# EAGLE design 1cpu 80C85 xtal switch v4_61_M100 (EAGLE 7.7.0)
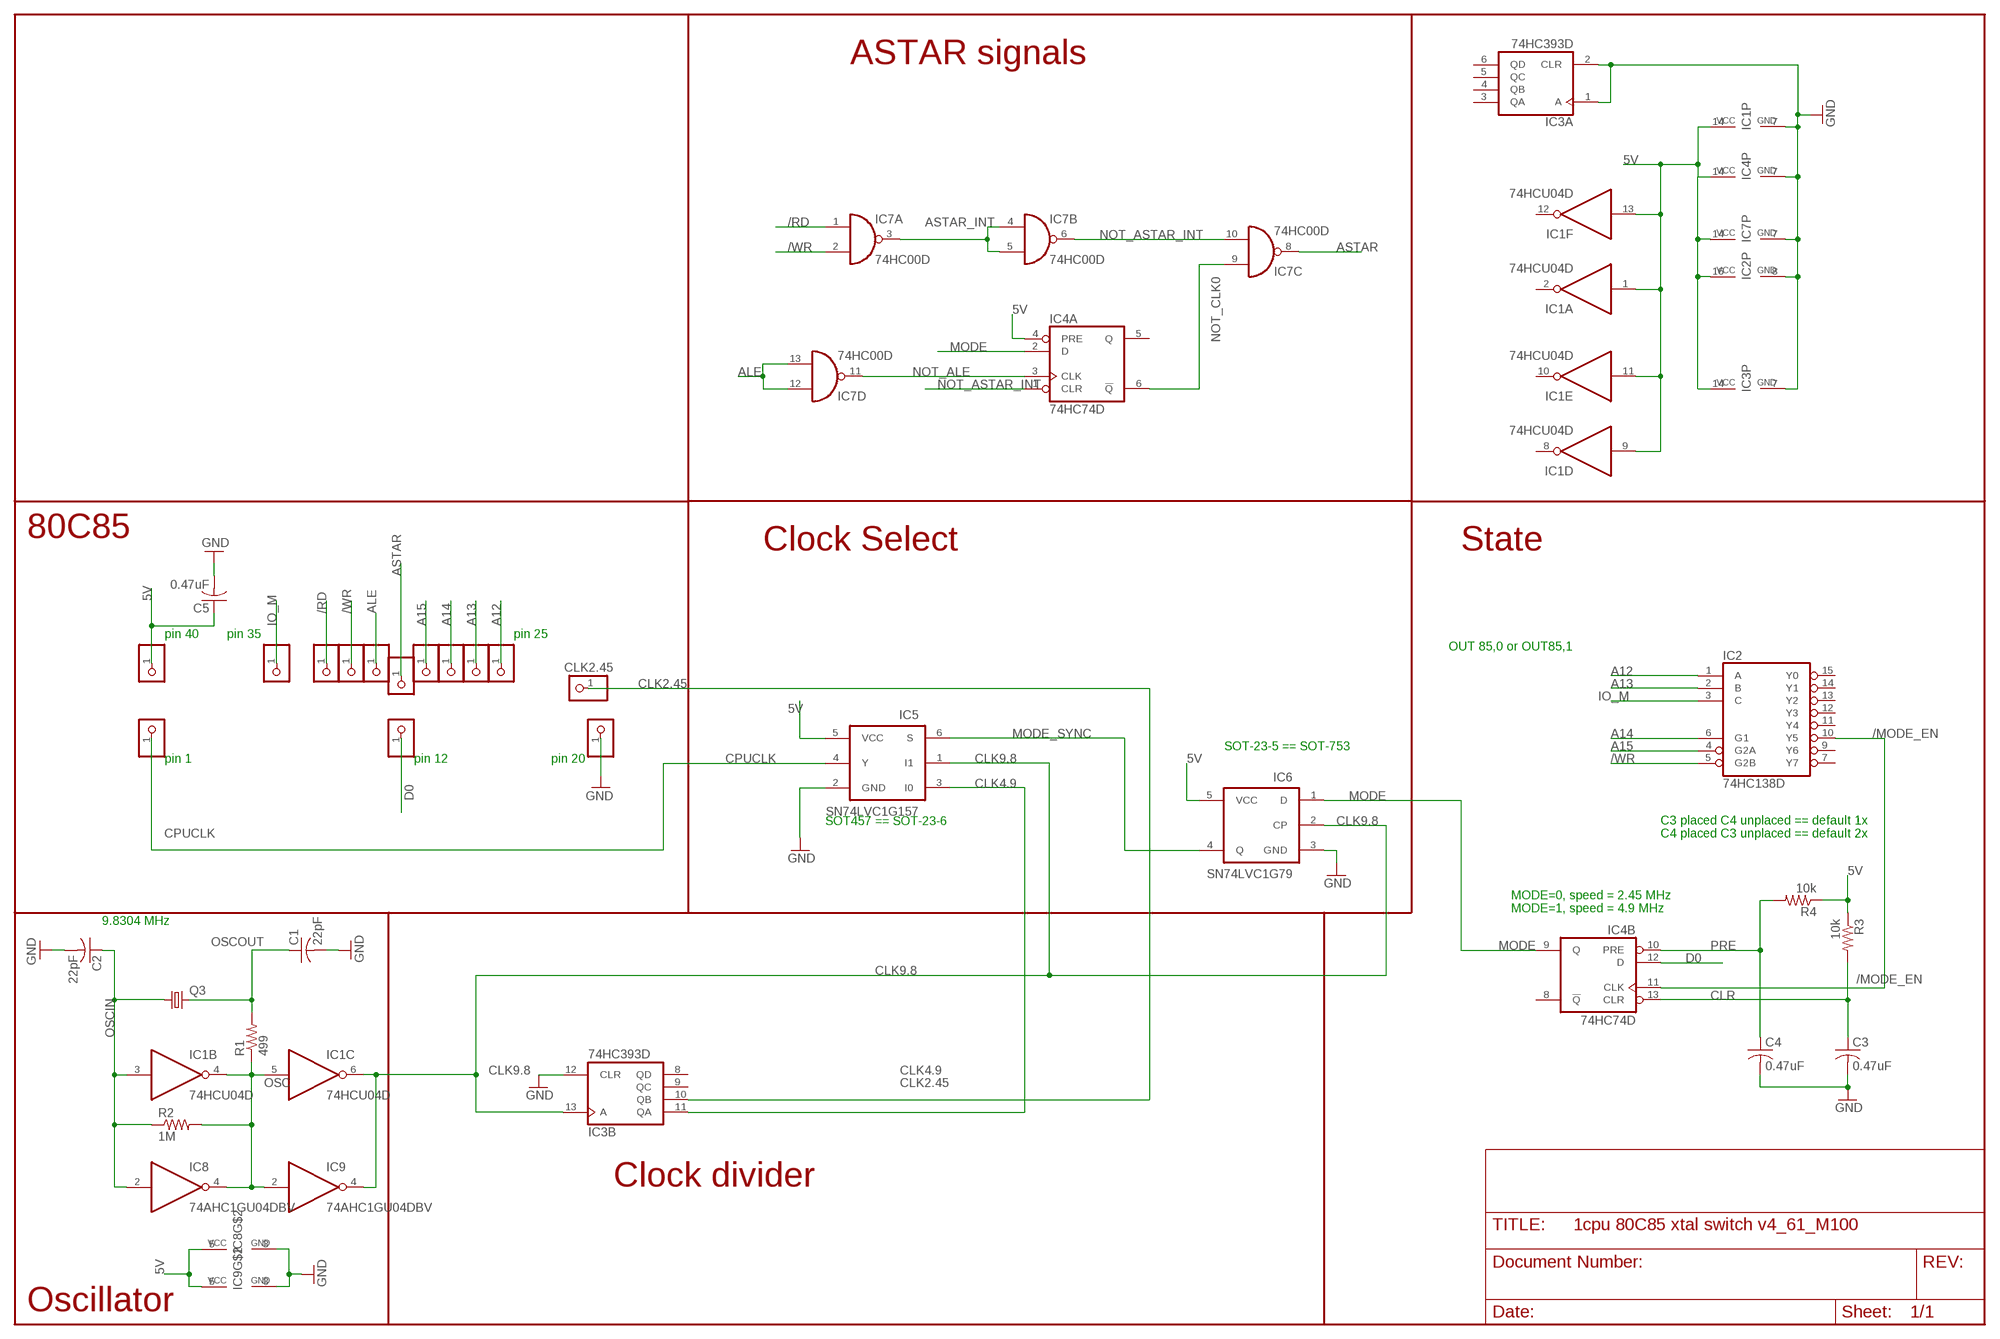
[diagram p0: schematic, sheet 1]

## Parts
5V  PINHD-1X1  [1X01]
5V1  PINHD-1X1  [1X01]
5V2  PINHD-1X1  [1X01]
5V3  PINHD-1X1  [1X01]
5V5  PINHD-1X1  [1X01]
5V7  PINHD-1X1  [1X01]
5V8  PINHD-1X1  [1X01]
5V9  PINHD-1X1  [1X01]
5V10  PINHD-1X1  [1X01]
C1  22pF  C-US025-025X050  [C025-025X050]
C2  22pF  C-US025-025X050  [C025-025X050]
C3  0.47uF  C-US025-025X050  [C025-025X050]
C4  0.47uF  C-US025-025X050  [C025-025X050]
C5  0.47uF  C-US025-025X050  [C025-025X050]
GND5  PINHD-1X1  [1X01]
GND8  PINHD-1X1  [1X01]
GND10  PINHD-1X1  [1X01]
IC1  74HCU04D  74HC04D  [SO14]
IC2  74HC138D  [SO16]
IC3  74HC393D  [SO14]
IC4  74HC74D  [SO14]
IC5  SN74LVC1G157  [SOT23-6]
IC6  SN74LVC1G79  [SOT23-5]
IC7  74HC00D  [SO14]
IC8  74AHC1GU04DBV  [SOT23-5]
IC9  74AHC1GU04DBV  [SOT23-5]
Q3  CRYSTALHC49S  [HC49/S]
R1  499  R-US_0204/5  [0204/5]
R2  1M  R-US_0204/5  [0204/5]
R3  10k  R-US_0204/5  [0204/5]
R4  10k  R-US_0204/5  [0204/5]
SEL2  PINHD-1X1  [1X01]
SEL3  PINHD-1X1  [1X01]

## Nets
5V: 5V.1 C5.1 IC1.1(A:I) IC1.9(D:I) IC1.11(E:I) IC1.13(F:I) IC1.14(P:VCC) IC2.16(VCC) IC3.14(P:VCC) IC4.4(A:PRE) IC4.14(P:VCC) IC5.5(VCC) IC6.5(VCC) IC7.14(P:VCC) IC8.5(VCC) IC9.5(VCC) R3.1 R4.1
/MODE_EN: IC2.10(Y5) IC4.11(B:CLK)
/RD: 5V5.1 IC7.1(A:I0)
/WR: 5V3.1 IC2.5(G2B) IC7.2(A:I1)
A12: 5V10.1 IC2.1(A)
A13: 5V9.1 IC2.2(B)
A14: 5V8.1 IC2.6(G1)
A15: 5V7.1 IC2.4(G2A)
ALE: GND10.1 IC7.12(D:I0) IC7.13(D:I1)
ASTAR: IC7.8(C:O) SEL3.1
ASTAR_INT: IC7.3(A:O) IC7.4(B:I0) IC7.5(B:I1)
CLK2.45: IC3.10(B:QB) SEL2.1
CLK4.9: IC3.11(B:QA) IC5.3(I0)
CLK9.8: IC1.6(C:O) IC3.13(B:A) IC5.1(I1) IC6.2(CP) IC9.4(O)
CLR: C3.1 IC4.13(B:CLR) R3.2
CPUCLK: 5V2.1 IC5.4(Y)
D0: GND8.1 IC4.12(B:D)
GND: C1.2 C2.2 C3.2 C4.2 C5.2 GND5.1 IC1.7(P:GND) IC2.8(GND) IC3.1(A:A) IC3.2(A:CLR) IC3.7(P:GND) IC3.12(B:CLR) IC4.7(P:GND) IC5.2(GND) IC6.3(GND) IC7.7(P:GND) IC8.3(GND) IC9.3(GND)
IO_M: 5V1.1 IC2.3(C)
MODE: IC4.2(A:D) IC4.9(B:Q) IC6.1(D)
MODE_SYNC: IC5.6(S) IC6.4(Q)
NOT_ALE: IC4.3(A:CLK) IC7.11(D:O)
NOT_ASTAR_INT: IC4.1(A:CLR) IC7.6(B:O) IC7.10(C:I1)
NOT_CLK0: IC4.6(A:!Q) IC7.9(C:I0)
OSC: IC1.4(B:O) IC1.5(C:I) IC8.4(O) IC9.2(I) R1.1 R2.2
OSCIN: C2.1 IC1.3(B:I) IC8.2(I) Q3.1 R2.1
OSCOUT: C1.1 Q3.2 R1.2
PRE: C4.1 IC4.10(B:PRE) R4.2
Unconnected: IC1.2(A:O) IC1.8(D:O) IC1.10(E:O) IC1.12(F:O) IC2.7(Y7) IC2.9(Y6) IC2.11(Y4) IC2.12(Y3) IC2.13(Y2) IC2.14(Y1) IC2.15(Y0) IC3.3(A:QA) IC3.4(A:QB) IC3.5(A:QC) IC3.6(A:QD) IC3.8(B:QD) IC3.9(B:QC) IC4.5(A:Q) IC4.8(B:!Q)

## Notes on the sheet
- ASTAR signals
- 80C85
- Clock Select | State
- pin 40 | pin 35 | pin 25
- OUT 85,0 or OUT85,1
- SOT-23-5 == SOT-753
- pin 1 | pin 12 | pin 20
- SOT457 == SOT-23-6
- C3 placed C4 unplaced == default 1x
  C4 placed C3 unplaced == default 2x
- MODE=0, speed = 2.45 MHz
  MODE=1, speed = 4.9 MHz
- 9.8304 MHz
- Clock divider
- Oscillator

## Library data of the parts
5V 5V1-5V3 5V5 5V7-5V10 GND5 GND8 GND10 SEL2 SEL3 = pinhead:PINHD-1X1: PIN HEADER
C1-C5 = resistor:C-US: CAPACITOR, American symbol
IC1 = 74xx-eu:74*04: Hex INVERTER
IC2 = 74xx-eu:74*138: 3-line to 8-line DECODER/DEMULTIPLEXER
IC3 = 74xx-eu:74*393: Dual 4-bit decade and binary COUNTER
IC4 = 74xx-eu:74*74: Dual D type positive edge triggered FLIP FLOP, preset and clear
IC5 = 74LV:SN74LVC1G157: SINGLE 2-INPUT MULTIPLEXER
IC6 = 74LV:SN74LVC1G79: D-TYPE FLIP-FLOP
IC7 = 74xx-eu:74*00: Quad 2-input NAND gate
IC8 IC9 = 74xx-little-us:74*1GU04: Single Unbuffered Inverter
Q3 = crystal:CRYSTAL: CRYSTAL; OC_FARNELL: 1667008; OC_NEWARK: unknown
R1-R4 = resistor:R-US_: RESISTOR, American symbol

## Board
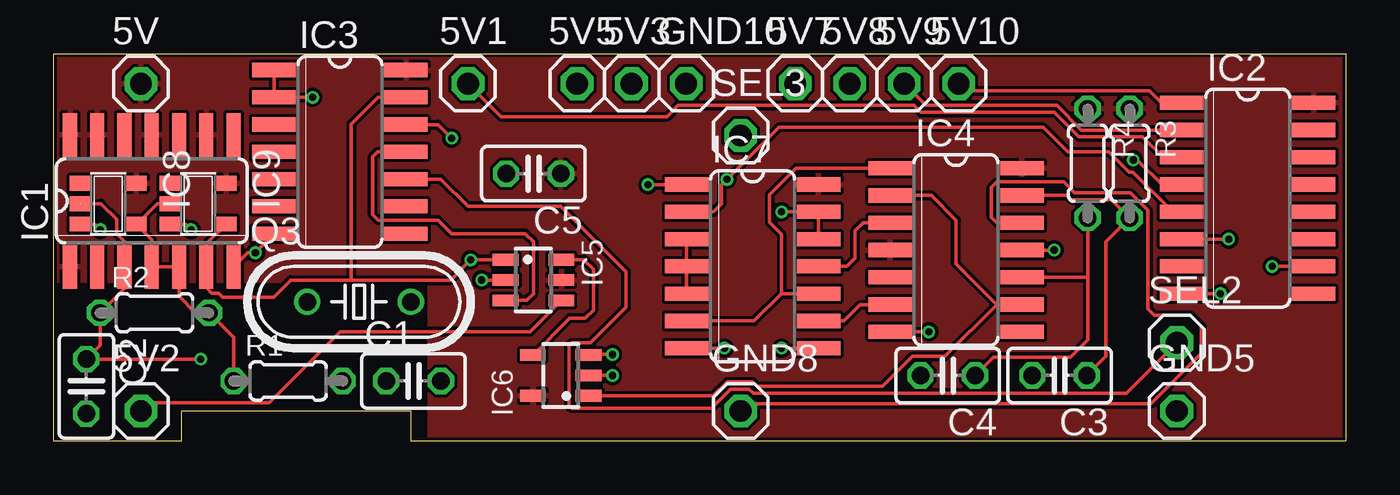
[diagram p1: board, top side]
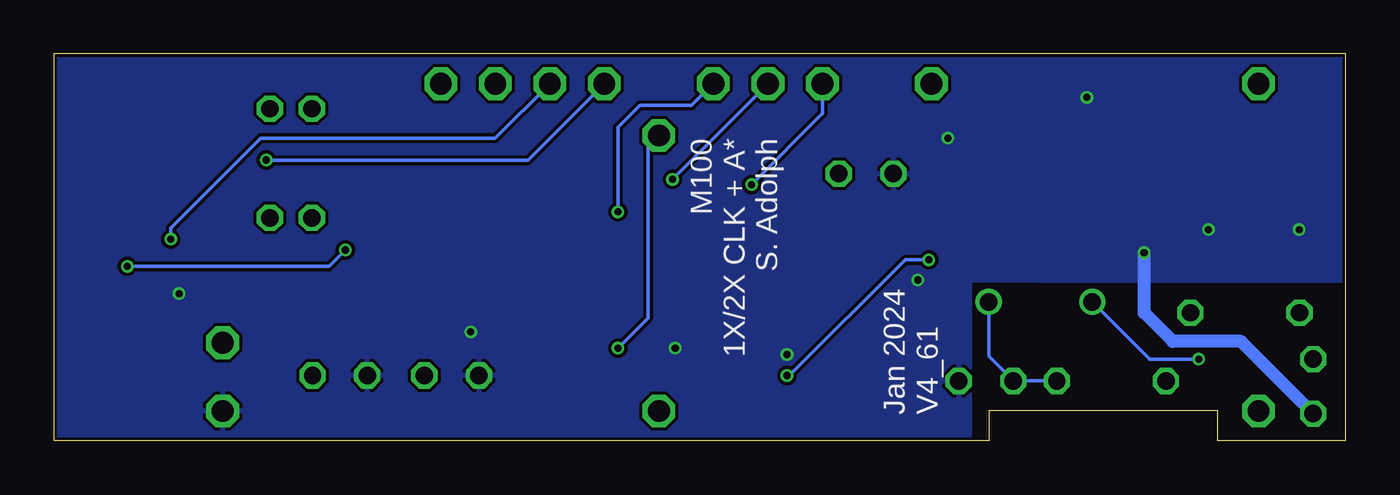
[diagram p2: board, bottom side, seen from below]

Size 60.2 x 18.03 mm. Coordinates in mm from the lower left corner, seen from the top.
Outline: 0,0 5.97,0 5.97,1.4 16.64,1.4 16.64,0 60.2,0 60.2,18.03 0,18.03 0,0
Copper layers (1*16): Top 0.035559375mm / dielectric 1.6mm / Bottom 0.035559375mm
Design rules "oshpark-2layer *": minimum track width 6mil, minimum drill 10mil, track to track 6mil, track to pad 6mil, pad to pad 6mil, via to via 6mil, smd to smd 6mil, copper to edge 6mil, drill to drill 6mil, minimum pad ring 5mil, minimum via ring 5mil, stop-mask expansion 2.5mil, vias tented up to drill 0mil, thermal gap 6mil

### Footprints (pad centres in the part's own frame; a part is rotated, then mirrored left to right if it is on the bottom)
1X01 = drill 1.016 octagon: 1 0,0
C025-025X050 = drill 0.813 octagon: 1 -1.27,0; 2 1.27,0
SO14 = smd 0.66 x 2.032: 1 -3.81,-3.073; 2 -2.54,-3.073; 3 -1.27,-3.073; 4 0,-3.073; 5 1.27,-3.073; 6 2.54,-3.073; 7 3.81,-3.073; 8 3.81,3.073; 9 2.54,3.073; 10 1.27,3.073; 11 0,3.073; 12 -1.27,3.073; 13 -2.54,3.073; 14 -3.81,3.073
SO16 = smd 0.66 x 2.032: 1 -4.445,-3.073; 2 -3.175,-3.073; 3 -1.905,-3.073; 4 -0.635,-3.073; 5 0.635,-3.073; 6 1.905,-3.073; 7 3.175,-3.073; 8 4.445,-3.073; 9 4.445,3.073; 10 3.175,3.073; 11 1.905,3.073; 12 0.635,3.073; 13 -0.635,3.073; 14 -1.905,3.073; 15 -3.175,3.073; 16 -4.445,3.073
SOT23-6 = smd 0.55 x 1.2: 1 -0.95,-1.3; 2 0,-1.3; 3 0.95,-1.3; 4 0.95,1.3; 5 0,1.3; 6 -0.95,1.3
SOT23-5 = smd 0.55 x 1.2: 1 -0.95,-1.3; 2 0,-1.3; 3 0.95,-1.3; 4 0.95,1.3; 5 -0.95,1.3
SOT23-5' = smd 0.69 x 0.99: 1 -0.95,-1.29; 2 0,-1.29; 3 0.95,-1.29; 4 0.95,1.3; 5 -0.95,1.3
HC49/S = drill 0.813: 1 -2.413,0; 2 2.413,0
0204/5 = drill 0.813 octagon: 1 -2.54,0; 2 2.54,0

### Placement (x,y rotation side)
5V  4.06,16.64 0 top
5V1  19.3,16.64 0 top
5V2  4.06,1.4 0 top
5V3  26.92,16.64 0 top
5V5  24.38,16.64 0 top
5V7  34.54,16.64 0 top
5V8  37.08,16.64 0 top
5V9  39.62,16.64 0 top
5V10  42.16,16.64 0 top
C1  16.76,2.79 0 top
C2  1.52,2.54 270 top
C3  46.86,3.05 180 top
C4  41.66,3.05 180 top
C5  22.35,12.45 180 top
GND5  52.32,1.4 0 top
GND8  32,1.4 0 top
GND10  29.46,16.64 0 top
IC1  4.57,11.18 0 top
IC2  55.63,11.3 270 top
IC3  13.34,13.46 270 top
IC4  42.04,8.89 270 top
IC5  22.35,7.49 270 top
IC6  23.62,3.05 90 top
IC7  32.56,8.13 270 top
IC8  74AHC1GU04DBV  [SOT23-5']  2.54,11.05 270 top
IC9  74AHC1GU04DBV  [SOT23-5']  6.73,11.05 270 top
Q3  14.22,6.48 0 top
R1  10.92,2.79 0 top
R2  4.7,5.97 0 top
R3  50.13,12.93 270 top
R4  48.17,12.93 270 top
SEL2  52.32,4.57 0 top
SEL3  32,14.22 0 top

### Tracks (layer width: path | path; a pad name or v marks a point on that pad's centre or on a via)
5V
  pour Top: 0.06,17.95 0.08,7.44 17.5,7.44 17.49,0.08 60.12,0.09 60.12,17.96
/MODE_EN  (via drill 0.33)
  Top 0.152: IC2.10 v56.77,8.13 | IC4.11 v46.61,8.89
  Bottom 0.152: v56.77,8.13 47.37,8.13 v46.61,8.89
/RD  (via drill 0.33)
  Top 0.152: v27.69,11.94 IC7.1
  Bottom 0.152: 5V5.1 24.38,15.23 24.4,15.23 v27.69,11.94
/WR  (via drill 0.33)
  Top 0.152: 28.68,10.67 IC7.2 30.73,10.67 31.11,11.05 31.11,11.93 v31.37,12.18 33.8,14.61 46.1,14.61 47.24,13.46 49.16,13.46 50.1,12.52 50.28,12.52 52.13,10.67 IC2.5
  Bottom 0.152: 5V3.1 26.92,16.62 v31.37,12.18
A12
  Top 0.152: 5V10.1 42.49,16.31 51.05,16.31 51.61,15.75 IC2.1
A13
  Top 0.152: IC2.2 47.88,14.48 46.74,15.62 40.64,15.62 5V9.1
A14  (via drill 0.33)
  Top 0.152: v54.74,9.4 IC2.6
  Bottom 0.152: 5V8.1 39.62,14.1 50.55,14.1 54.74,9.91 v54.74,9.4
A15  (via drill 0.33)
  Top 0.152: IC2.4 51.64,11.94 50.5,13.08 v50.29,13.08
  Bottom 0.152: 5V7.1 38.1,13.08 v50.29,13.08
ALE  (via drill 0.33)
  Top 0.152: IC7.12 IC7.13 v33.91,10.67
  Bottom 0.152: v33.91,10.67 33.91,14.61 32.89,15.62 30.48,15.62 GND10.1
ASTAR  (via drill 0.33)
  Top 0.152: 33.9,4.32 v33.91,4.32 IC7.8
  Bottom 0.152: SEL3.1 32.51,13.72 32.51,5.71 v33.91,4.32
ASTAR_INT
  Top 0.152: IC7.3 IC7.4 IC7.5
CLK2.45
  Top 0.152: SEL2.1 49.96,2.21 32.6,2.21 32.4,2.41 31.53,2.41 30.64,1.52 24.13,1.52 24,1.65 24,4.45 24.13,4.57 25.02,4.57 26.67,6.22 26.67,7.87 23.62,10.92 19.3,10.92 18.03,12.19 IC3.10
CLK4.9
  Top 0.152: IC5.3 22.04,6.54 22.35,6.86 22.35,9.27 21.97,9.65 18.54,9.65 17.91,10.29 15.11,10.29 14.86,10.54 14.86,13.23 15.09,13.46 IC3.11
CLK9.8  (via drill 0.33)
  Top 0.152: 13.87,7.49 11.05,7.49 10.25,6.69 7.87,6.69 7.68,6.88 7.37,6.88 7.1,7.15 7.1,8.09 IC1.6 7.11,9.18 IC9.4 | 13.87,7.49 18.49,7.49 v19.43,8.43 19.44,8.44 IC5.1 | IC6.2 v26.04,3.05 | 13.87,7.49 13.87,14.76 15.11,16 IC3.13
  Bottom 0.152: v19.43,8.43 20.52,8.43 25.91,3.05 v26.04,3.05
CLR
  Top 0.152: IC4.13 47.23,11.43 47.42,11.24 49.28,11.24 R3.2 49.02,9.28 49.02,3.94 C3.1
CPUCLK
  Top 0.152: 5V2.1 4.45,1.78 10.03,1.78 13.35,5.09 22.2,5.09 IC5.4
D0
  Top 0.152: GND8.1 32.33,1.73 51.12,1.73 53.47,4.08 53.47,5.33 52.96,5.84 51.27,5.84 50.97,6.15 50.97,10.74 50.15,11.56 47.56,11.56 47.05,12.06 43.94,12.06 43.69,11.81 43.69,10.41 43.94,10.16 IC4.12
GND  (via drill 0.33)
  Top 0.152: IC4.7 v40.77,5.08 | IC7.7 v31.24,4.32 | IC2.8 v54.36,6.86 | IC1.7 9.04,8.76 v9.4,8.76 10.26,9.63 | IC3.1 IC3.2 v12.07,16 | IC5.2 v19.94,7.49 | IC6.3 24.89,4.03 v26.04,4.03 | IC3.12 17.91,14.73 v18.54,14.1 | IC8.3 1.91,10.1 v2.17,9.84 | IC9.3 6.14,10.1 v6.4,9.84
  Top 0.406: 10.26,9.63 IC3.7
  Bottom 0.152: v31.24,4.32 31.41,4.32 31.41,4.33 | v54.36,6.86 54.47,6.86
  Bottom 0.61: C2.2 4.89,4.64 8.06,4.64 9.4,5.97 v9.4,8.76
  pour Bottom: 0.06,17.95 60.12,17.96 60.12,0.09 17.49,0.08 17.5,7.45 14.3,7.44 0.08,7.44 0.08,11.63
IO_M
  Top 0.152: 5V1.1 20.84,15.1 28.56,15.1 29.08,15.62 40.06,15.62 40.07,15.63 40.4,15.3 46.62,15.3 47.75,14.17 50.72,14.17 51.69,13.21 IC2.3
MODE
  Top 0.152: IC4.9 43.94,6.35 | 43.94,6.35 42.04,8.26 42.04,10.29 40.89,11.43 IC4.2 | IC6.1 30.72,2.1 31.38,2.76 32.56,2.76 32.77,2.55 38.62,2.55 40,3.94 41.53,3.94 43.94,6.35
MODE_SYNC
  Top 0.152: IC5.6 24.69,8.44 25.15,7.99 25.15,6.1 24.77,5.71 24.04,5.71 IC6.4 | IC6.4
NOT_ALE
  Top 0.152: IC7.11 36.96,8.13 37.34,8.51 37.34,9.78 37.72,10.16 IC4.3
NOT_ASTAR_INT
  Top 0.152: IC7.6 32.63,5.59 33.9,6.86 | 33.9,6.86 IC7.10 | IC4.1 34.58,12.7 33.35,11.47 33.35,10.17 33.9,9.63 33.9,6.86
NOT_CLK0
  Top 0.152: IC4.6 38.95,6.34 37.57,6.34 36.82,5.59 IC7.9
OSC
  Top 0.152: R1.1 8.38,4.83 R2.2 6.6,5.97 5.84,6.73 IC1.5 IC1.4 4.57,9.37 IC8.4 3.86,10.1 4.81,11.05 IC9.2
OSCIN  (via drill 0.33)
  Top 0.152: v6.86,3.81 C2.1 2.17,4.46 R2.1 3.3,7.11 IC1.3 3.3,9.28 2.93,9.65 2.93,10.31 2.2,11.05 IC8.2
  Bottom 0.152: Q3.1 9.16,3.82 9.16,3.81 v6.86,3.81
OSCOUT
  Bottom 0.152: R1.2 C1.1 16.64,3.94 Q3.2
PRE
  Top 0.152: C4.1 43.78,3.9 47.36,3.9 48.17,4.71 48.17,7.59 | R4.2 48.17,7.59 | IC4.10 48.15,7.62 48.17,7.59

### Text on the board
_tsilk: A* | +5 | IO/M | /RD | /WR | ALE | A15 | A14 | A13 | A12 | U04 | U04 | C5 | 74HC393 | R4 | R3 | 74HC138 | 74HC74 | R2 | 1G157 | 74HC00 | C2 | 2.45M | D0 | C4 | C3 | 1 | R1 | 1G79 | 2X | 1X | GND | C1
_bsilk: M100 / 1X/2X CLK + A* / S. Adolph | Jan 2024 / V4_61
